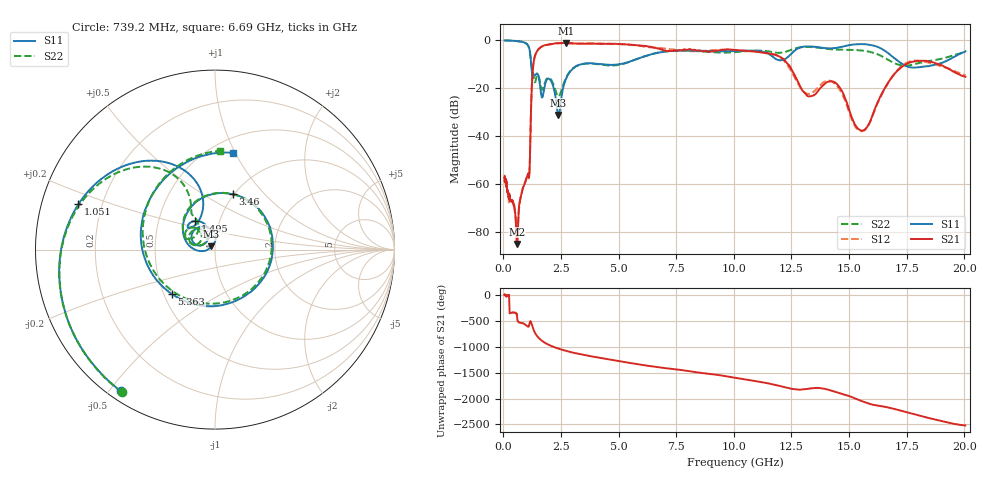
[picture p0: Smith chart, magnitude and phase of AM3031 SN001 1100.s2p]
# Hz S DB R 50
!freq MagS11 AngS11 MagS21 AngS21 MagS12 AngS12 MagS22 AngS22
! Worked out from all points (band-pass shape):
!   1601 points, 50 MHz to 20.05 GHz, reference 50 ohm
!   highest |S21| = -1.04 dB at 2.702 GHz (marker M1); lowest = -85.1 dB at 581.6 MHz (marker M2)
!   |S21| within 3 dB of the highest: 1.492 GHz to 6.919 GHz (5.427 GHz wide, 129 % of centre); 9.405 GHz to 10.11 GHz (706.3 MHz wide, 7.24 % of centre)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
!   lowest |S11| = -31.2 dB at 2.388 GHz (marker M3), VSWR 1.06, Z = 48 + j1.87 ohm
!   |S11| at or under -10 dB: 1.203 GHz to 3.355 GHz (2.152 GHz wide, 94.4 % of centre); 4.305 GHz to 4.994 GHz (689 MHz wide, 14.8 % of centre); 17.34 GHz to 18.81 GHz (1.472 GHz wide, 8.14 % of centre)
!   |S22| runs from -23.4 to 0.0 dB; largest |S21 - S12| = 0.068
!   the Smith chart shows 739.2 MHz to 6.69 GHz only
!   S11 on the Smith chart (normalised r, x): 739.2 MHz: 0.04, -0.54; 1.051 GHz: 0.11, +0.16; 1.495 GHz: 0.77, +0.25; 3.46 GHz: 0.99, +0.68; 5.363 GHz: 0.55, -0.31; 6.69 GHz: 0.64, +0.98
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5e7  -0.04 -8.1  -58.78 -5.5  -56.13 1.8  -0.05 -8.1
1.35947e8  -0.07 -21.7  -60.77 -19.3  -61.10 -17.9  -0.06 -21.6
3.696318e8  -0.14 -58.8  -67.12 16.6  -66.98 18.3  -0.14 -59.3
5.816099e8  -0.29 -94.7  -85.07 -25.8  -85.62 -48.7  -0.27 -94.7
7.39193e8  -0.48 -123.5  -65.76 178.1  -65.79 178.4  -0.46 -123.2
1.005007e9  -1.44 176.0  -57.54 124.1  -57.15 123.2  -1.42 177.5
1.051217e9  -1.92 161.7  -56.00 109.2  -55.80 106.4  -1.92 163.5
1.494952e9  -14.26 124.3  -3.99 -94.4  -4.01 -95.1  -14.39 143.7
1.769459e9  -19.90 166.1  -2.11 163.1  -2.14 162.6  -18.56 166.0
2.387798e9  -31.19 135.2  -1.19 42.5  -1.19 42.4  -23.45 142.6
2.702015e9  -16.34 169.3  -1.04 0.4  -1.21 0.4  -15.84 161.5
2.722335e9  -15.89 166.6  -1.05 -2.2  -1.21 -2.2  -15.44 159.8
3.459926e9  -9.80 72.4  -1.44 -76.8  -1.27 -75.3  -9.85 77.1
5.363178e9  -9.25 -134.0  -1.71 134.8  -1.71 134.9  -9.34 -145.2
6.689795e9  -5.21 79.2  -3.40 43.0  -3.14 46.9  -5.16 87.1
7.401857e9  -4.33 9.9  -4.28 7.7  -3.95 3.4  -4.33 26.6
8.76102e9  -4.41 -108.7  -4.43 -75.9  -4.38 -72.9  -4.73 -93.0
1.056581e10  -4.27 83.5  -4.46 164.0  -4.40 164.9  -4.51 79.9
1.293477e10  -2.82 -102.7  -20.33 -26.7  -20.31 -18.4  -2.82 -94.5
1.554104e10  -1.55 68.0  -37.71 112.2  -37.96 116.0  -4.23 80.7
1.725979e10  -9.53 -59.9  -11.33 -74.7  -10.94 -71.6  -10.40 -95.1
2.005e10  -4.63 69.4  -15.21 1.0  -14.55 3.0  -4.93 79.8
